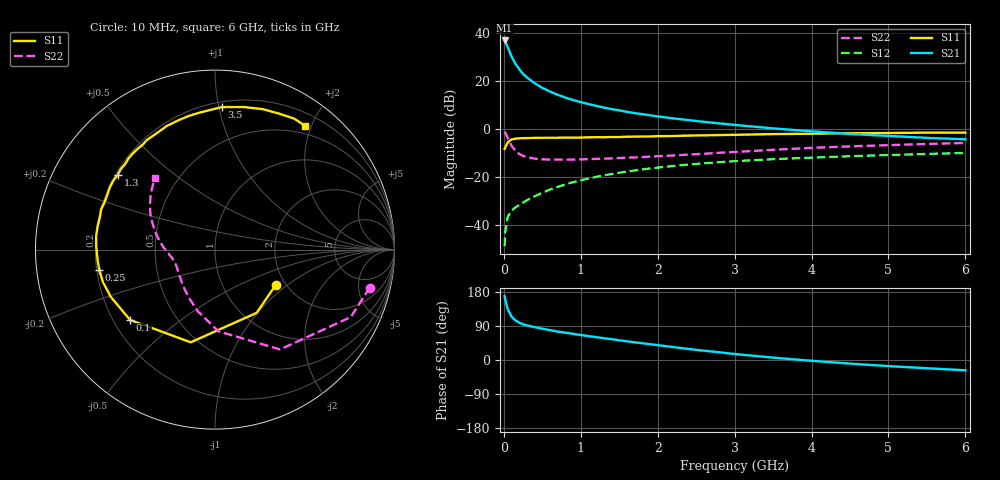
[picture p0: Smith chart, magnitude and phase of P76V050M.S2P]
! SIEMENS Small Signal Semiconductors
! BFP196
! Si NPN RF Bipolar Junction Transistor in SOT143
! VCE = 6 V  IC = 50 mA
! Common Emitter S-Parameters:  May  1996
# GHz  S  MA  R  50
!  f  S11  S21  S12  S22
! GHz  MAG  ANG  MAG  ANG  MAG  ANG  MAG  ANG
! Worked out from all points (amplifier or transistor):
!   36 points, 10 MHz to 6 GHz, reference 50 ohm
!   highest |S21| = 37.0 dB at 10 MHz (marker M1)
!   |S21| within 3 dB of that: start of sweep to 52.78 MHz
!   unconditionally stable (mu >= 1): 489.6 MHz to 4.456 GHz
!   at 250 MHz: K = 0.81, MSG = 26.8 dB, |S12| = -30.5 dB
!   at 1.4 GHz: K = 1.08, MAG = 11.7 dB, |S12| = -18.6 dB
!   at 6 GHz: K = 0.97, MSG = 2.8 dB, |S12| = -9.8 dB
!   S11 on the Smith chart (normalised r, x): 10 MHz: 1.77, -0.83; 100 MHz: 0.27, -0.34; 250 MHz: 0.21, -0.08; 1.3 GHz: 0.21, +0.33; 3.5 GHz: 0.24, +1.02; 6 GHz: 0.38, +1.91
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0.01  0.3914 -30.4  70.56 168.7  0.0037 80.5  0.8876 -13.8
0.02  0.4219 -56.6  66.11 157.6  0.0076 74.2  0.8449 -26.4
0.05  0.5341 -104.7  51.22 134.4  0.0151 56.3  0.664 -56.9
0.1  0.6145 -140.4  32.66 114.4  0.0202 48.4  0.456 -87.5
0.15  0.6377 -155.6  23.15 104.6  0.0237 48.1  0.3574 -105.5
0.2  0.6501 -164.0  17.79 98.5  0.0267 50.0  0.3077 -117.7
0.25  0.6547 -170.2  14.29 94.4  0.0299 52.7  0.2792 -127.1
0.3  0.6566 -174.5  12.01 91.4  0.0334 54.9  0.264 -133.6
0.4  0.6625 178.2  9.104 86.7  0.0404 57.8  0.2457 -143.5
0.5  0.6666 173.5  7.289 82.6  0.0477 59.9  0.2377 -150.1
0.6  0.6667 168.5  6.082 78.8  0.0557 61.1  0.2343 -154.5
0.7  0.6667 164.0  5.23 75.0  0.0633 61.3  0.2339 -158.0
0.9  0.6698 156.7  4.07 69.0  0.0796 60.6  0.2345 -163.2
1.1  0.681 149.3  3.345 63.0  0.0947 59.3  0.2396 -166.7
1.3  0.6828 142.5  2.836 57.4  0.1103 57.0  0.2449 -169.8
1.7  0.7051 130.2  2.173 46.6  0.139 52.0  0.2598 -175.5
2.2  0.7251 116.7  1.688 34.2  0.1726 44.8  0.2849 177.9
2.8  0.7585 101.3  1.329 20.4  0.2073 36.2  0.3247 168.4
3.5  0.7952 87.2  1.044 6.3  0.2388 26.3  0.3743 157.9
4.5  0.8269 71.1  0.801 -9.6  0.2755 14.5  0.4412 145.2
5.5  0.8526 58.8  0.663 -21.8  0.3075 3.8  0.4956 134.7
6  0.853 53.8  0.619 -27.1  0.3224 -1.8  0.5209 129.7
